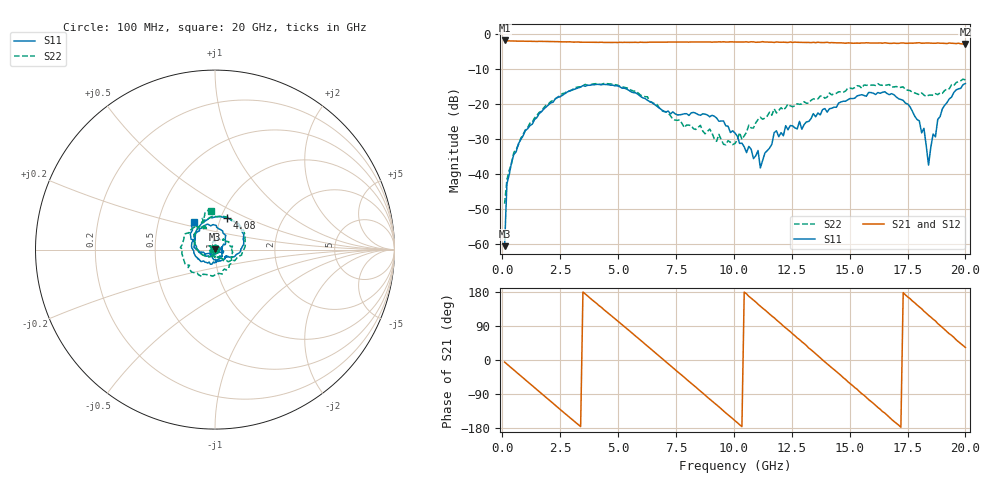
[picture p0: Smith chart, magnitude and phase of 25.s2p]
!Agilent Technologies,N5230C,MY49001569,A.09.33.09
!Agilent N5230C: A.09.33.09
!Date: Monday, July 27, 2015 10:36:07
!Correction: S11(Full 2 Port(1,2))
!S21(Full 2 Port(1,2))
!S12(Full 2 Port(1,2))
!S22(Full 2 Port(1,2))
!S2P File: Measurements: S11, S21, S12, S22:
# Hz S  dB  R 50
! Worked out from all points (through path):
!   201 points, 100 MHz to 20 GHz, reference 50 ohm
!   highest |S21| = -1.96 dB at 100 MHz (marker M1); lowest = -3.0 dB at 20 GHz (marker M2)
!   group delay of S21, straight-line fit = 145 ps
!   lowest |S11| = -60.5 dB at 100 MHz (marker M3), VSWR 1.00, Z = 50 + j0.0928 ohm
!   |S11| at or under -10 dB: start of sweep to end of sweep
!   |S22| runs from -48.5 to -13.0 dB; largest |S21 - S12| = 0.023
!   S11 on the Smith chart (normalised r, x): 100 MHz: 1.00, +0.00; 4.08 GHz: 1.07, +0.39; 20 GHz: 0.75, +0.24
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1e8  -60.54 98.6  -1.96 -5.5  -1.97 -5.7  -48.46 89.9
1.995e8  -42.77 -15.6  -2.07 -10.9  -2.08 -10.8  -41.63 -41.8
6.97e8  -31.38 -90.9  -2.15 -36.8  -2.16 -36.8  -31.67 -93.1
1.9905e9  -20.31 -179.5  -2.27 -104.0  -2.27 -104.0  -20.04 179.7
3.483e9  -14.82 98.7  -2.45 179.3  -2.48 179.1  -14.80 97.6
4.08e9  -14.45 69.2  -2.53 149.0  -2.48 148.8  -14.25 68.4
5.3735e9  -15.80 10.1  -2.51 82.9  -2.53 82.8  -15.47 5.9
6.7665e9  -21.15 -28.2  -2.44 10.9  -2.41 10.9  -21.04 -43.4
7.5625e9  -23.16 -33.9  -2.40 -30.6  -2.40 -30.4  -24.71 -55.9
8.458e9  -23.07 -50.9  -2.38 -77.1  -2.46 -76.9  -26.70 -73.2
1.005e10  -28.35 -131.1  -2.38 -160.4  -2.38 -160.2  -31.31 156.3
1.1045e10  -33.31 93.6  -2.44 147.3  -2.46 147.1  -24.49 77.0
1.11445e10  -38.26 95.0  -2.42 142.1  -2.36 142.5  -23.82 74.3
1.1841e10  -27.69 17.7  -2.38 105.8  -2.45 105.3  -22.61 36.1
1.3433e10  -22.79 -86.6  -2.49 21.8  -2.51 21.7  -18.60 -40.5
1.4229e10  -21.26 -124.3  -2.56 -20.5  -2.61 -20.7  -17.46 -80.4
1.51245e10  -18.52 -176.1  -2.74 -67.4  -2.48 -67.1  -15.72 -126.8
1.67165e10  -17.41 100.3  -2.78 -151.0  -2.75 -150.9  -14.51 152.0
1.8209e10  -26.99 -17.5  -2.70 128.8  -2.83 129.2  -17.50 113.2
1.8408e10  -37.46 -52.2  -2.68 118.0  -2.72 118.6  -17.56 114.6
1.9005e10  -21.44 -171.1  -2.75 85.9  -2.73 86.0  -17.01 114.0
2e10  -14.24 127.8  -2.97 33.1  -2.92 31.7  -13.20 95.7
